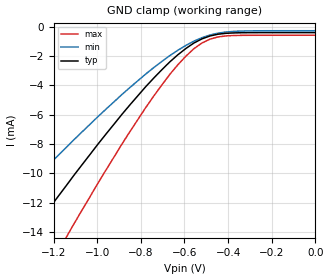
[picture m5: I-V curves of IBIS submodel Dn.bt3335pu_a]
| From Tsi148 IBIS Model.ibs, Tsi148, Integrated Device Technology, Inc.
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[Submodel]  Dn.bt3335pu_a
Submodel_type   Dynamic_clamp
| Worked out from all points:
|   GND clamp passes 1 mA (typ) near -0.54 V on its own axis
[GND Clamp]   | Note: Vtable =  Vout
| Voltage   I(typ)   I(min)   I(max)
-3.6V     -65.12mA   -49.03mA   -83.81mA
-1.51V    -18.39mA   -13.85mA   -24.16mA
-1.29V    -13.81mA   -10.44mA   -18.24mA
-1.143V   -10.86mA   -8.244mA   -14.39mA
-1.107V   -10.13mA   -7.707mA   -13.45mA
-887mV    -5.975mA   -4.621mA   -8.006mA
-777mV    -4.072mA   -3.212mA   -5.492mA
-667mV    -2.387mA   -1.958mA   -3.238mA
-557mV    -1.105mA   -975uA     -1.492mA
-483mV    -622uA     -556uA     -838uA
-410mV    -441uA     -352uA     -618uA
0V        -392uA     -264uA     -571uA
